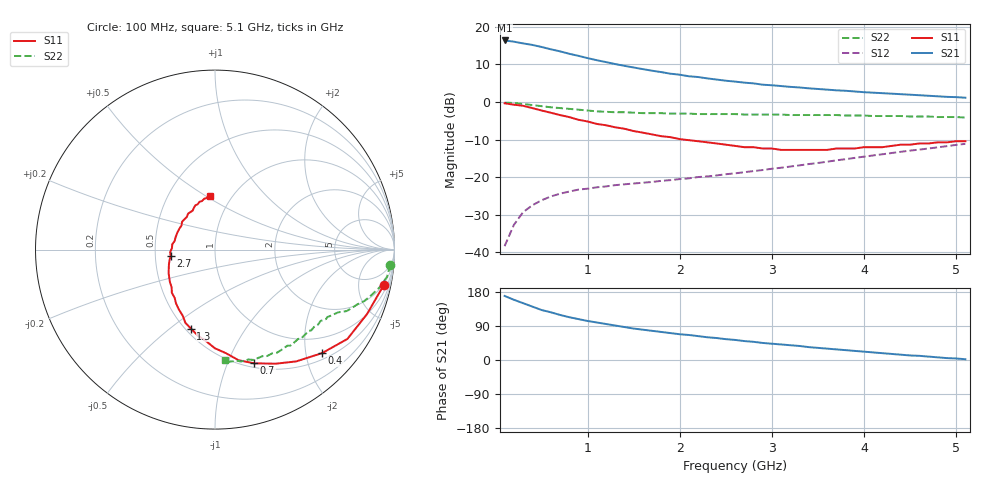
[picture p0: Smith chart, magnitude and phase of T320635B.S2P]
!AT-32063
!S AND NOISE PARAMETERS per side at Vce=5 V  Ic=2mA.  LAST UPDATED 11-11-96
# ghz s ma r 50
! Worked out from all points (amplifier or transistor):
!   51 points, 100 MHz to 5.1 GHz, reference 50 ohm
!   highest |S21| = 16.4 dB at 100 MHz (marker M1)
!   |S21| within 3 dB of that: start of sweep to 716.4 MHz
!   unconditionally stable (mu >= 1): 1.713 GHz to 4.211 GHz
!   at 900 MHz: K = 0.60, MSG = 17.8 dB, |S12| = -23.3 dB
!   at 2.6 GHz: K = 1.14, MAG = 10.0 dB, |S12| = -19.0 dB
!   at 5.1 GHz: K = 0.89, MSG = 6.1 dB, |S12| = -11.2 dB
!   lowest NFmin = 0.75 dB at 900 MHz
!   S11 on the Smith chart (normalised r, x): 100 MHz: 1.80, -9.16; 400 MHz: 0.63, -2.33; 700 MHz: 0.54, -1.25; 1.3 GHz: 0.53, -0.59; 2.7 GHz: 0.60, -0.04; 5.1 GHz: 0.80, +0.52
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0.1  0.96 -12.0  6.6 169.0  0.012 83.0  0.98 -5.0
0.2  0.92 -23.0  6.36 159.0  0.023 76.0  0.97 -9.0
0.3  0.89 -34.0  6.03 150.0  0.034 70.0  0.94 -13.0
0.4  0.83 -44.0  5.76 141.0  0.042 65.0  0.91 -16.0
0.5  0.77 -54.0  5.41 132.0  0.049 60.0  0.88 -19.0
0.7  0.67 -71.0  4.73 119.0  0.06 53.0  0.83 -23.0
0.8  0.63 -78.0  4.39 113.0  0.064 51.0  0.81 -25.0
0.9  0.58 -84.0  4.12 108.0  0.068 50.0  0.79 -26.0
1  0.55 -90.0  3.84 103.0  0.07 48.0  0.77 -27.0
1.1  0.51 -96.0  3.6 99.0  0.073 47.0  0.75 -29.0
1.3  0.46 -107.0  3.2 91.0  0.078 46.0  0.73 -31.0
1.5  0.41 -116.0  2.88 83.0  0.082 46.0  0.72 -33.0
1.8  0.35 -130.0  2.5 74.0  0.089 47.0  0.71 -36.0
2  0.32 -139.0  2.31 68.0  0.094 48.0  0.7 -39.0
2.2  0.3 -148.0  2.15 63.0  0.1 49.0  0.69 -41.0
2.5  0.27 -162.0  1.92 55.0  0.109 51.0  0.69 -44.0
2.6  0.26 -167.0  1.87 53.0  0.112 51.0  0.69 -46.0
2.7  0.25 -172.0  1.81 50.0  0.116 52.0  0.68 -47.0
2.9  0.24 178.0  1.7 45.0  0.124 52.0  0.68 -49.0
3.5  0.23 149.0  1.49 32.0  0.154 53.0  0.67 -57.0
4.3  0.26 117.0  1.29 16.0  0.209 50.0  0.65 -69.0
5.1  0.3 95.0  1.14 2.0  0.277 44.0  0.62 -85.0
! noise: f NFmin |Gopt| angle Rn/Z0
0.9  0.75  0.74  47  0.37
1.8  1.26  0.55  101  0.22
2.4  1.6  0.45  139  0.13
